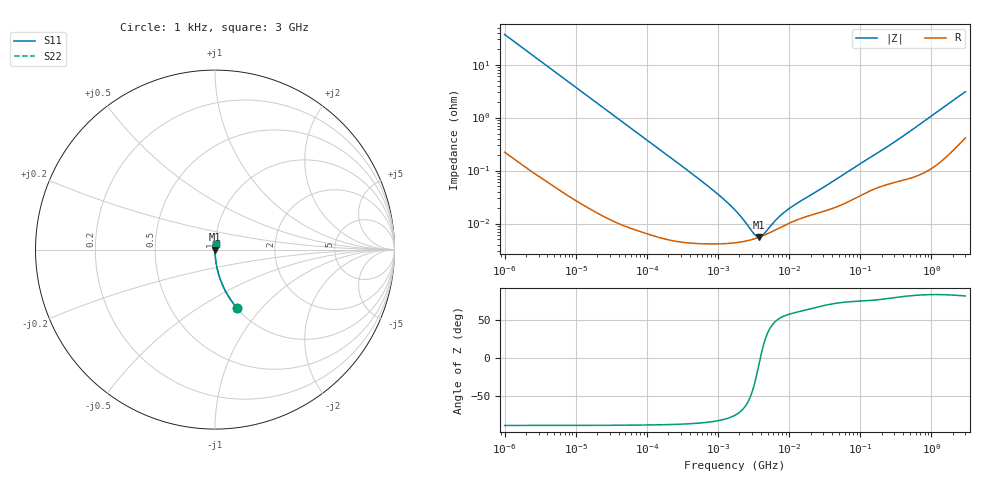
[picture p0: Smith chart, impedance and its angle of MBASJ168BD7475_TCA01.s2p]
! MBASJ168BD7475_TCA01  S-PARAMETER MODEL  ( Standard Model )
! Model Generated by TAIYO YUDEN Corporation (http://www.ty-top.com)
! Version 1.0
! TAIYO YUDEN Control No. 240819
! Copyright(c) 2024 TAIYO YUDEN CO.,LTD. All Rights Reserved.
! Product Description (link to TY-COMPAS)
! https://ds.yuden.co.jp/TYCOMPAS/or/detail?pn=MBASJ168BD7475KTCA01&u=M
! Products Name : Multilayer Ceramic Capacitors
! Characteristics :
!  Capacitance : 4.7 [uF] , Rated Voltage : 6.3 [V] , TCC : X7T
!  Case Size : 1.6 x 0.8 / 0.063 x 0.031 [mm/inch] , Thickness : 0.8 / 0.031 [mm/inch]
!  (Conditions: Temperature = 25 [degC] , DC Bias Voltage = 0 [V])
! External Node Assignments :
!  1  o---| |---o  2
! GND o---------o GND
! Frequency Range : 1kHz  -  3GHz  [ 401 STEP ]
# MHZ S RI R 50
! Freq[MHz].  S11 Real  S11 Imag  S21 Real  S21 Imag  S12 Real  S12 Imag  S22 Real  S22 Imag
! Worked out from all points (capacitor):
!   401 points, 1 kHz to 3 GHz, reference 50 ohm
!   read as one part in series: C = 4.29 uF near 1.077 kHz
!   lowest |Z| = 5.56 mohm at 3.79 MHz (marker M1)
!   series resonance near 3.934 MHz, so ESL is about 380 pH
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0.001  0.1222 -0.3246  0.8778 0.3246  0.8778 0.3246  0.1222 -0.3246
0.001685  0.0475 -0.2096  0.9525 0.2096  0.9525 0.2096  0.0475 -0.2096
0.00306  0.0153 -0.1196  0.9847 0.1196  0.9847 0.1196  0.0153 -0.1196
0.005768  0.00459 -0.0644  0.9954 0.0644  0.9954 0.0644  0.00459 -0.0644
0.01216  0.00118 -0.0307  0.9988 0.0307  0.9988 0.0307  0.00118 -0.0307
0.147855  6.1e-05 -0.00256  0.9999 0.00256  0.9999 0.00256  6.1e-05 -0.00256
0.791611  4.14e-05 -0.000459  1 0.000459  1 0.000459  4.14e-05 -0.000459
1.238299  4.18e-05 -0.000275  1 0.000275  1 0.000275  4.18e-05 -0.000275
1.732051  4.32e-05 -0.000175  1 0.000175  1 0.000175  4.32e-05 -0.000175
2.334012  4.59e-05 -0.000103  1 0.000103  1 0.000103  4.59e-05 -0.000103
2.514714  4.69e-05 -8.7e-05  1 8.7e-05  1 8.7e-05  4.69e-05 -8.7e-05
2.709407  4.8e-05 -7.15e-05  1 7.15e-05  1 7.15e-05  4.8e-05 -7.15e-05
3.789741  5.51e-05 -6.82e-06  0.9999 6.82e-06  0.9999 6.82e-06  5.51e-05 -6.82e-06
5.502215  6.84e-05 5.92e-05  0.9999 -5.92e-05  0.9999 -5.92e-05  6.84e-05 5.92e-05
5.928204  7.18e-05 7.21e-05  0.9999 -7.21e-05  0.9999 -7.21e-05  7.18e-05 7.21e-05
7.988506  8.77e-05 0.000123  0.9999 -0.000123  0.9999 -0.000123  8.77e-05 0.000123
9.991309  0.000101 0.000162  0.9999 -0.000162  0.9999 -0.000162  0.000101 0.000162
21.06097  0.000146 0.000327  0.9999 -0.000327  0.9999 -0.000327  0.000146 0.000327
256.0921  0.000567 0.00293  0.9994 -0.00293  0.9994 -0.00293  0.000567 0.00293
501.0334  0.000742 0.00547  0.9993 -0.00547  0.9993 -0.00547  0.000742 0.00547
2226.275  0.00326 0.023  0.9967 -0.023  0.9967 -0.023  0.00326 0.023
3000  0.00499 0.0301  0.995 -0.0301  0.995 -0.0301  0.00499 0.0301
